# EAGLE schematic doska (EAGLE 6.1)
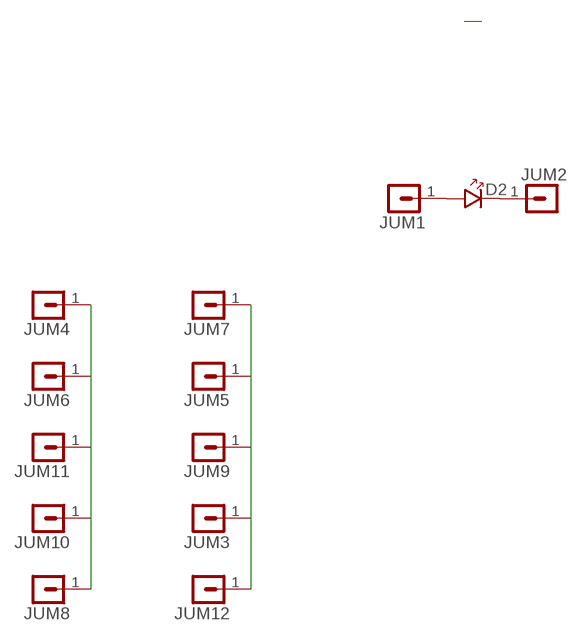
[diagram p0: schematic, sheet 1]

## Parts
D2  LED_5  [LED_5]
JUM1  S1G1_JUMP  [S1G1_JUM]
JUM2  S1G1_JUMP  [S1G1_JUM]
JUM3  S1G1_JUMP  [S1G1_JUM]
JUM4  S1G1_JUMP  [S1G1_JUM]
JUM5  S1G1_JUMP  [S1G1_JUM]
JUM6  S1G1_JUMP  [S1G1_JUM]
JUM7  S1G1_JUMP  [S1G1_JUM]
JUM8  S1G1_JUMP  [S1G1_JUM]
JUM9  S1G1_JUMP  [S1G1_JUM]
JUM10  S1G1_JUMP  [S1G1_JUM]
JUM11  S1G1_JUMP  [S1G1_JUM]
JUM12  S1G1_JUMP  [S1G1_JUM]

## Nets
N$1: D2.A JUM1.1
N$2: D2.K JUM2.1
N$4: JUM4.1 JUM6.1 JUM8.1 JUM10.1 JUM11.1
N$5: JUM3.1 JUM5.1 JUM7.1 JUM9.1 JUM12.1

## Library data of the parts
D2 = #PaJa_30:LED: LED - jednobarevna
JUM1-JUM12 = #PaJa_konektory:S1G1_JUMP: Radove konektory - koliky - 1x

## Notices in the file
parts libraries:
Copyright (C) PaJa 2001-2011
Copyright (C) PaJa 2011
